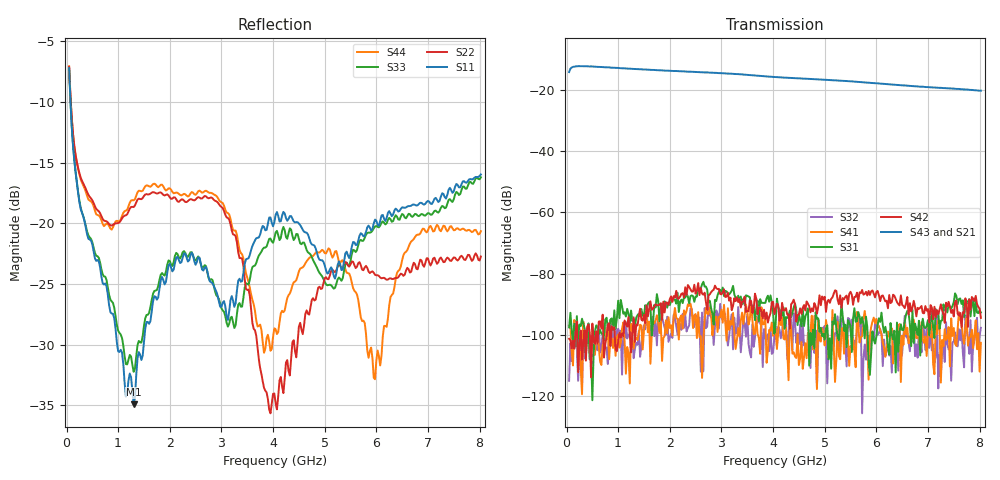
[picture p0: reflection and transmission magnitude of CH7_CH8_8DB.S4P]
!Agilent Technologies,E5071C,MY46316741,A.11.02
!Date: Mon Jun 01 10:28:53 2026
!Data & Calibration Information:
!1:CH7 INPUT 2:CH7 OUTPUT 3:CH8 INPUT 4:CH8 OUTPUT
!Freq	S11:SOLT4(ON)	S12:SOLT4(ON)	S13:SOLT4(ON)	S14:SOLT4(ON)
!	S21:SOLT4(ON)	S22:SOLT4(ON)	S23:SOLT4(ON)	S24:SOLT4(ON)
!	S31:SOLT4(ON)	S32:SOLT4(ON)	S33:SOLT4(ON)	S34:SOLT4(ON)
!	S41:SOLT4(ON)	S42:SOLT4(ON)	S43:SOLT4(ON)	S44:SOLT4(ON)
!PortZ  Port1:50+j0  Port2:50+j0  Port3:50+j0  Port4:50+j0
!Above PortZ is port z conversion or system Z0 setting when saving the data.
!When reading, reference impedance value at option line is always used.
# Hz S dB R 50
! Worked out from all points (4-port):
!   320 points, 50 MHz to 8.025 GHz, reference 50 ohm
!   strongest paths, dB at 50 MHz, 2.05 GHz, 4.05 GHz, 6.05 GHz, 8.025 GHz:
!     S43: -14.1, -13.8, -15.8, -17.9, -20.2
!     S21: -14.2, -13.8, -15.9, -18.1, -20.4
!     S42: -101.3, -89.3, -91.6, -87.1, -94.5
!     S31: -97.6, -88.5, -96.5, -94.6, -92.7
!     S41: -97.0, -100.3, -98.0, -97.1, -102.7
!     S32: -115.1, -101.1, -97.2, -99.5, -97.7
!   lowest |S11| = -34.9 dB at 1.3 GHz (marker M1), VSWR 1.04, Z = 48.6 - j1.13 ohm
!   |S11| at or under -10 dB: 77.05 MHz to end of sweep
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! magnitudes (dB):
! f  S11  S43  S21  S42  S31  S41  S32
! 50 MHz  -7.2  -14.1  -14.2  -101.3  -97.6  -97.0  -115.1
! 1.3 GHz  -34.9  -13.1  -13.2  -94.3  -94.9  -104.6  -107.7
! 2 GHz  -23.3  -13.7  -13.8  -88.4  -90.3  -97.8  -100.9
! 3.025 GHz  -26.5  -14.5  -14.6  -86.1  -84.6  -96.1  -95.1
! 3.95 GHz  -19.5  -15.7  -15.8  -93.0  -87.2  -98.7  -97.7
! 5.275 GHz  -23.1  -16.9  -17.1  -90.1  -101.8  -107.0  -99.5
! 8.025 GHz  -16.0  -20.2  -20.4  -94.5  -92.7  -102.7  -97.7
